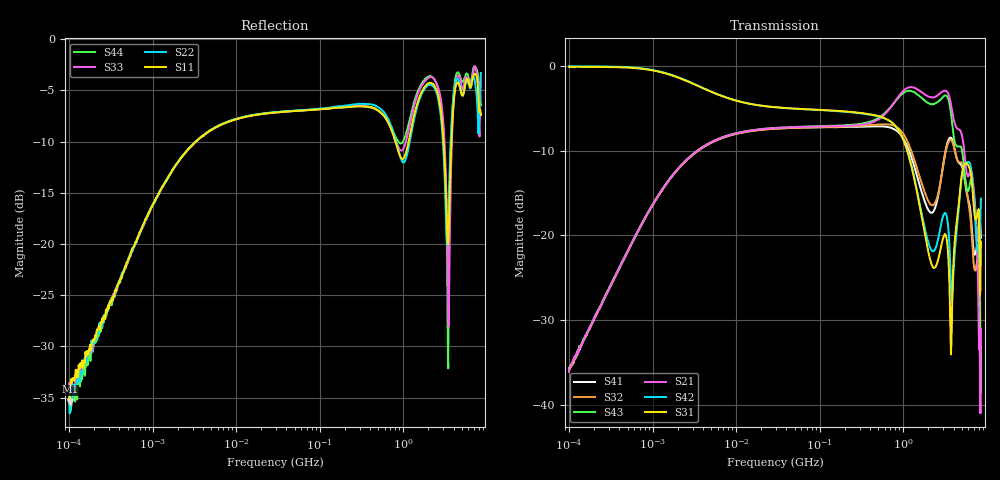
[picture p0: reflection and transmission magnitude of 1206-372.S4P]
!Agilent Technologies,E5071C,MY46110495,A.10.06
!Date: Tue Jun 06 11:40:34 2017
!Data & Calibration Information:
!Freq	S11:SOLT4(ON)	S12:SOLT4(ON)	S13:SOLT4(ON)	S14:SOLT4(ON)
!	S21:SOLT4(ON)	S22:SOLT4(ON)	S23:SOLT4(ON)	S24:SOLT4(ON)
!	S31:SOLT4(ON)	S32:SOLT4(ON)	S33:SOLT4(ON)	S34:SOLT4(ON)
!	S41:SOLT4(ON)	S42:SOLT4(ON)	S43:SOLT4(ON)	S44:SOLT4(ON)
!PortZ  Port1:50+j0  Port2:50+j0  Port3:50+j0  Port4:50+j0
!Above PortZ is port z conversion or system Z0 setting when saving the data.
!When reading, reference impedance value at option line is always used.
# Hz S dB R 50
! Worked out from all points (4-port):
!   801 points, 100 kHz to 8.5 GHz, reference 50 ohm
!   strongest paths, dB at 100 kHz, 1.721 MHz, 29.51 MHz, 502.3 MHz, 8.5 GHz:
!     S31: -0.1, -1.2, -4.9, -5.9, -20.7
!     S42: -0.1, -1.1, -4.9, -6.0, -15.7
!     S21: -36.1, -13.0, -7.4, -6.3, -31.0
!     S43: -35.6, -12.9, -7.3, -6.2, -33.2
!     S32: -35.7, -13.0, -7.4, -6.9, -36.1
!     S41: -35.9, -13.0, -7.4, -7.2, -20.3
!   lowest |S11| = -35.4 dB at 101.7 kHz (marker M1), VSWR 1.03, Z = 51.1 + j1.33 ohm
!   |S11| at or under -10 dB: start of sweep to 3.307 MHz; 802.9 MHz to 1.158 GHz (355.5 MHz wide, 36.2 % of centre); 3.035 GHz to 3.778 GHz (742.7 MHz wide, 21.8 % of centre)
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100000  -35.03 56.8  -35.77 88.0  -0.12 -0.8  -35.99 -91.6
        -36.07 88.5  -35.36 68.0  -35.96 -95.1  -0.09 -0.7
        -0.13 -0.8  -35.68 -93.5  -33.61 69.0  -35.69 86.8
        -35.86 -91.6  -0.06 -0.9  -35.59 86.5  -34.81 76.5
101665  -35.42 50.1  -35.41 89.6  -0.13 -0.8  -35.58 -92.7
        -35.50 88.0  -36.54 71.1  -35.68 -91.1  -0.09 -0.8
        -0.13 -0.8  -35.70 -93.4  -34.83 67.4  -35.51 90.1
        -35.62 -91.1  -0.07 -0.9  -35.55 86.6  -35.43 74.1
4165418  -9.34 32.2  -9.49 32.5  -2.73 -14.5  -9.54 -148.0
         -9.49 32.6  -9.30 32.5  -9.52 -148.0  -2.72 -14.7
         -2.74 -14.6  -9.53 -147.8  -9.31 32.2  -9.48 32.6
         -9.52 -147.9  -2.71 -14.7  -9.46 32.5  -9.30 32.7
1.216903e9  -9.14 70.5  -2.53 2.6  -11.35 -113.5  -10.45 62.0
            -2.53 2.6  -9.63 69.5  -9.76 60.4  -11.28 -114.6
            -11.35 -113.4  -9.76 60.5  -8.09 67.4  -2.98 -2.2
            -10.43 62.1  -11.27 -114.6  -2.97 -2.2  -7.54 67.2
4.638388e9  -4.42 -113.5  -7.50 -46.6  -16.11 94.8  -11.47 -51.0
            -7.51 -46.5  -4.09 -115.9  -11.42 -53.8  -16.61 86.0
            -16.11 94.9  -11.42 -53.6  -3.59 -109.9  -9.56 -45.7
            -11.46 -50.9  -16.62 86.0  -9.55 -45.7  -3.34 -105.3
6.738951e9  -3.94 14.1  -13.16 -67.0  -14.55 -13.8  -20.19 137.4
            -13.12 -67.0  -3.92 10.1  -21.26 137.1  -13.65 -17.8
            -14.55 -13.5  -21.28 137.2  -3.64 13.8  -13.91 -56.1
            -20.18 137.7  -13.65 -17.5  -13.88 -55.9  -3.31 14.3
8.5e9  -7.40 109.8  -30.88 79.7  -20.68 34.4  -20.26 35.8
       -31.00 79.8  -3.30 125.3  -35.96 140.1  -15.68 16.8
       -20.73 34.5  -36.05 139.4  -3.78 127.8  -33.23 87.5
       -20.29 36.1  -15.66 17.2  -33.22 87.9  -6.50 96.3
